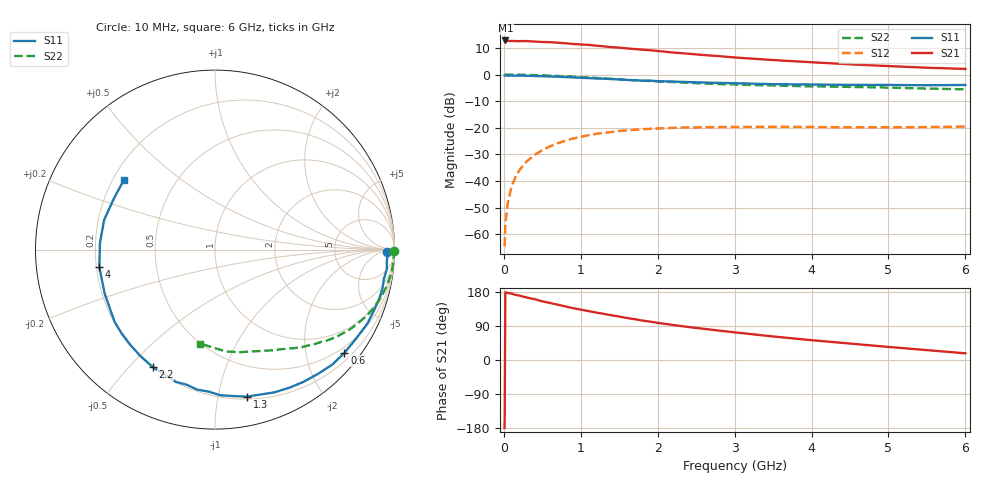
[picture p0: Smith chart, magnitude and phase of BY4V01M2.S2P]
! SIEMENS Small Signal Semiconductors
! BFY420
! Si NPN RF SIEGET Grounded Emitter Transistor in MICRO-X
! VCE = 4 V  IC = 1.2 mA
! Common Emitter S-Parameters:  October  1996
# GHz  S  MA  R  50
!  f  S11  S21  S12  S22
! GHz  MAG  ANG  MAG  ANG  MAG  ANG  MAG  ANG
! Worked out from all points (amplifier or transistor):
!   36 points, 10 MHz to 6 GHz, reference 50 ohm
!   highest |S21| = 12.8 dB at 20 MHz (marker M1)
!   |S21| within 3 dB of that: start of sweep to 1.607 GHz
!   unconditionally stable (mu >= 1): 4.384 GHz to end of sweep
!   at 250 MHz: K = 0.06, MSG = 23.4 dB, |S12| = -34.2 dB
!   at 1.4 GHz: K = 0.21, MSG = 15.9 dB, |S12| = -21.5 dB
!   at 6 GHz: K = 1.32, MAG = 7.4 dB, |S12| = -19.5 dB
!   S11 on the Smith chart (normalised r, x): 10 MHz: 46, -14; 600 MHz: 0.36, -2.81; 1.3 GHz: 0.22, -1.22; 2.2 GHz: 0.20, -0.58; 4 GHz: 0.21, -0.07; 6 GHz: 0.24, +0.32
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0.01  0.9607 -0.7  4.366 -179.5  0.0006 53.8  0.9997 -0.3
0.02  0.9641 -1.3  4.379 178.6  0.0016 80.0  0.9949 -0.6
0.05  0.9592 -3.4  4.269 176.9  0.0038 85.9  0.9975 -1.4
0.1  0.9634 -6.6  4.291 175.4  0.0079 85.5  0.9964 -2.9
0.15  0.955 -9.8  4.257 171.8  0.0118 83.1  0.9944 -4.4
0.2  0.9577 -13.0  4.25 170.1  0.0158 82.0  0.9938 -5.8
0.3  0.9508 -19.2  4.254 164.7  0.0236 78.5  0.9875 -8.7
0.4  0.9443 -25.8  4.173 160.5  0.0311 74.5  0.9798 -11.6
0.5  0.9298 -32.1  4.098 154.7  0.0381 71.1  0.9686 -14.4
0.6  0.9224 -38.6  4.06 150.5  0.0449 67.2  0.9571 -17.2
0.9  0.8864 -56.2  3.762 136.7  0.0632 56.9  0.9128 -24.8
1.1  0.861 -67.6  3.616 129.1  0.0728 50.9  0.8809 -29.5
1.3  0.8385 -77.7  3.393 121.7  0.0809 45.2  0.8475 -33.7
1.5  0.8121 -87.9  3.21 114.7  0.0871 40.4  0.8165 -37.6
1.8  0.7691 -101.8  2.94 104.1  0.0938 33.8  0.7715 -42.6
2.2  0.7406 -118.0  2.597 92.4  0.1001 26.5  0.7244 -48.8
2.8  0.6987 -138.2  2.221 77.5  0.1037 18.6  0.6643 -56.7
3.5  0.6618 -158.2  1.877 62.1  0.1048 12.5  0.6238 -64.7
4  0.6519 -171.3  1.706 52.3  0.1039 10.1  0.6019 -70.6
4.5  0.642 176.7  1.559 43.4  0.1027 8.1  0.5875 -76.7
5.5  0.6312 153.6  1.347 26.0  0.1037 8.0  0.5467 -90.9
6  0.6389 142.8  1.279 17.7  0.1056 9.1  0.5298 -98.9
